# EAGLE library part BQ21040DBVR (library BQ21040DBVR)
0.8A Single Input Single-Cell Li-Ion and Li-Pol Battery Charger Source: Datasheet
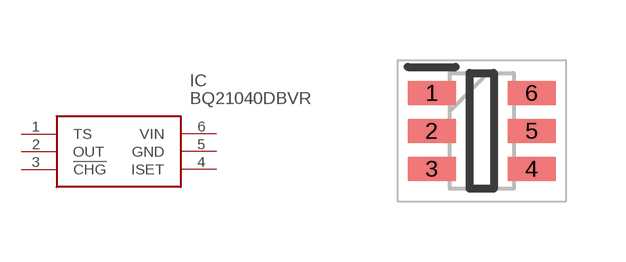
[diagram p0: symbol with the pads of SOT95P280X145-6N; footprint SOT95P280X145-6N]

Designator prefix IC

## BQ21040DBVR (Description: 0.8A Single Input Single-Cell Li-Ion and Li-Pol Battery Charger; Height: 1.45mm; Manufacturer_Name: Texas Instruments; Manufacturer_Part_Number: BQ21040DBVR; Mouser_Part_Number: 595-BQ21040DBVR; Mouser_Price-Stock: https://www.mouser.co.uk/ProductDetail/Texas-Instruments/BQ21040DBVR?qs=cttFivMKqWyovUuY6Xwwcw%3D%3D)  [SOT95P280X145-6N]
1  TS  in
2  OUT  out
3  !CHG  out
4  ISET  in
5  GND  pwr
6  VIN  in

## Footprint SOT95P280X145-6N (pad centres in mm)
DBV (R-PDSO-G6)
smd 1.2 x 0.6: 1 -1.25,0.95; 2 -1.25,0; 3 -1.25,-0.95; 4 1.25,-0.95; 5 1.25,0; 6 1.25,0.95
